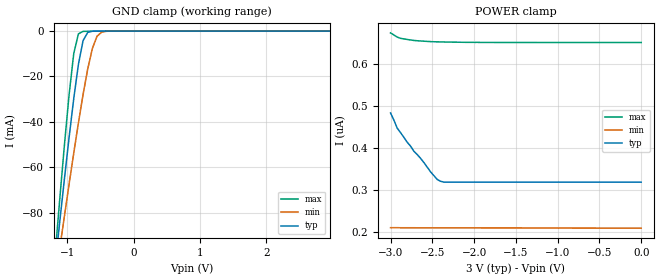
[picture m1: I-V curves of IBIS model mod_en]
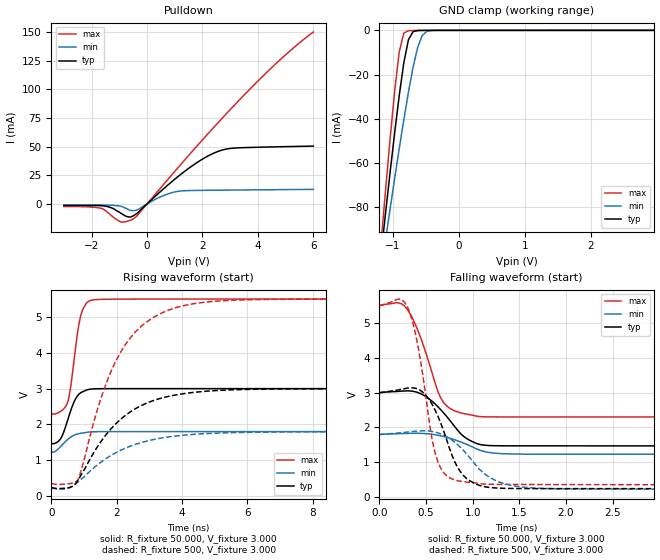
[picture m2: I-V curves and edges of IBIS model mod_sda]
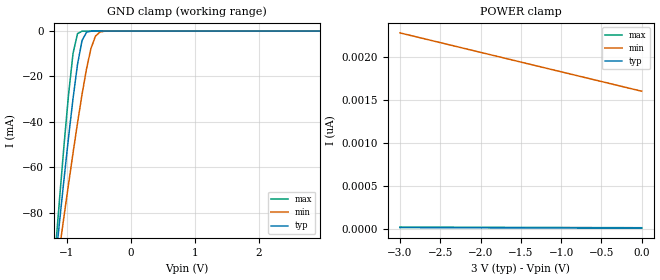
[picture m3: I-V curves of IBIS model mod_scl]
| IBIS (I/O, Buffer, Information, Specification) Model, officially
| electronic behavioral standard for Buffer structures of digital pins.
[IBIS ver]  4.0
[File name] m24c32_tssop8.ibs
[File Rev]  1.0
[Date]   5 April 2013
[Source]   CAD & Design Services (Catania) - STMicroelectronics
[Notes]
   (Note1)  This IBIS model includes the TSSOP8 package data
   (Note2)  This IBIS model has some Notes about the non-monotonicity
   of the I-V curves, but they are not indicative of problems
   inside the model;
[Copyright] (c) 2013 STMicroelectronics
|   Component M24C32
[Component] M24C32
[Manufacturer] STMicroelectronics
[Package]
| variable   typ   min   max
R_pkg   0.0   0.0   0.0
L_pkg   0.0H   0.0H   0.0H
C_pkg   0.0F   0.0F   0.0F
[Pin]  signal_name   model_name   R_pin   L_pin   C_pin
1   E0   mod_en   NA   NA   NA
2   E1   mod_en   NA   NA   NA
3   E2   mod_en   NA   NA   NA
4   VSS   GND   NA   NA   NA
5   SDA   mod_sda   NA   NA   NA
6   SCL   mod_scl   NA   NA   NA
7   WCN   mod_wcn   NA   NA   NA
8   VCC   POWER   NA   NA   NA
[Package Model]  182696_TSSOP8
[Define Package Model]  182696_TSSOP8
[Manufacturer]  STMicroelectronics
[OEM]  STMicroelectronics
[Description]  8 pin TSSOP package
[Number Of Pins]  8
[Pin Numbers]
|Pin Num   Terminal Name
1   | net1
2   | net2
3   | net3
4   | net4_GND
5   | net5
6   | net6
7   | net7
8   | net8_VDD
[Model Data]
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[End Model Data]
[End Package Model]
| Models and submodels in the file (4): mod_en (Input), mod_sda (I/O_open_drain), mod_scl (Input), mod_wcn (Input)
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|   Model mod_en
[Model]   mod_en
Model_type Input
Vinl   =   0.900V
Vinh   =   2.100V
C_comp   2.219pF   2.024pF   2.433pF
[Temperature Range]   25.0000   0.1250k   -40.0000
[Voltage Range]   3.0000V   1.8000V   5.5000V
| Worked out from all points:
|   GND clamp passes 1 mA (typ) near -0.70 V on its own axis
[GND_clamp]
|Voltage   I(typ)   I(min)   I(max)
-3V       -632.3mA   -502.5mA   -782.2mA
-1.18V    -103mA     -110.1mA   -98.28mA
-1.11V    -83.81mA   -95.65mA   -73.74mA
-1.04V    -65mA      -81.41mA   -50.04mA
-970mV    -46.81mA   -67.4mA    -27.99mA
-900mV    -29.69mA   -53.72mA   -9.875mA
-830mV    -14.68mA   -40.49mA   -1.207mA
-760mV    -4.236mA   -27.99mA   -124.1uA
-620mV    -70.96uA   -7.667mA   -43.96uA
-550mV    -18.49uA   -2.282mA   -30.81uA
-480mV    -9.663uA   -457.1uA   -18.98uA
2.95V     1.011uA    747.3nA    5.256uA
[POWER_clamp]
|Voltage   I(typ)   I(min)   I(max)
-3V       483.2nA    210.9nA    673.2nA
-2.92V    447.1nA    210.9nA    663.2nA
-2.8V     413.6nA    210.8nA    657.6nA
-2.76V    404.4nA    210.8nA    656.4nA
-2.72V    392.2nA    210.8nA    655.3nA
-2.68V    384.4nA    210.7nA    654.5nA
-2.6V     365.3nA    210.7nA    653.5nA
-2.52V    343.2nA    210.7nA    652.5nA
-2.44V    325.1nA    210.6nA    652nA
-2.4V     321nA      210.6nA    651.8nA
-2.36V    319nA      210.6nA    651.6nA
0V        319nA      209.8nA    650.4nA
|   Model mod_sda
[Model]   mod_sda
Model_type I/O_open_drain
Polarity   Non-Inverting
Enable   Active-High
Vinl   =   0.900V
Vinh   =   2.100V
Vmeas  =   1.500V
Cref   =   10pF
Rref   =   1k
Vref   =   3.000V
C_comp   2.925pF   2.793pF   3.207pF
[Temperature Range]   25.0000   0.1250k   -40.0000
[Voltage Range]   3.0000V   1.8000V   5.5000V
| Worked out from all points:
|   slope of the pulldown table from 0 to 0.45 V, typ, clamps not added: 44.7 ohm
|   GND clamp passes 1 mA (typ) near -0.70 V on its own axis
|   rising waveform, R_fixture 50.000, V_fixture 3.000: 20-80 % time 357ps typ, 419ps min, 284ps max; typ from 1.47 V to 3 V
|   rising waveform, R_fixture 500, V_fixture 3.000: 20-80 % time 1.55ns typ, 1.71ns min, 1.36ns max; typ from 0.243 V to 3 V
|   falling waveform, R_fixture 50.000, V_fixture 3.000: 20-80 % time 301ps typ, 316ps min, 241ps max; typ from 3 V to 1.47 V
|   falling waveform, R_fixture 500, V_fixture 3.000: 20-80 % time 247ps typ, 351ps min, 184ps max; typ from 3 V to 0.243 V
[Pulldown]
|Voltage   I(typ)   I(min)   I(max)
-3V       -1.423mA   -700uA     -2.3mA
-1.9V     -1.423mA   -747uA     -2.942mA
-1.5V     -1.922mA   -945.3uA   -5.832mA
-900mV    -8.724mA   -2.34mA    -15.92mA
-700mV    -11.22mA   -4.514mA   -15.11mA
-500mV    -10.4mA    -5.884mA   -13.16mA
900mV     19.57mA    9.89mA     25.58mA
1.8V      36.08mA    11.8mA     50.48mA
2.5V      45.28mA    12mA       69.26mA
3.1V      48.68mA    12.14mA    84.88mA
4.3V      49.66mA    12.4mA     114.4mA
6V        50.5mA     12.74mA    150mA
[GND_clamp]
|Voltage   I(typ)   I(min)   I(max)
-3V       -632.3mA   -502.5mA   -782.2mA
-1.18V    -103mA     -110.1mA   -98.29mA
-1.11V    -83.81mA   -95.65mA   -73.75mA
-1.04V    -65mA      -81.41mA   -50.05mA
-970mV    -46.82mA   -67.4mA    -28mA
-900mV    -29.7mA    -53.72mA   -9.899mA
-830mV    -14.69mA   -40.49mA   -1.245mA
-760mV    -4.25mA    -28mA      -159.3uA
-620mV    -83.69uA   -7.672mA   -65.52uA
-550mV    -26.12uA   -2.289mA   -45.81uA
-480mV    -12.79uA   -464.3uA   -27.85uA
2.95V     1.011uA    747.3nA    5.256uA
[Ramp]
| variable   typ   min   max
dV/dt_r  0.9163/0.4218n   0.3404/0.5426n   1.9194/0.3308n
dV/dt_f  0.9163/0.3279n   0.3404/0.3803n   1.9194/0.2635n
R_load = 50.0000
[Rising Waveform]
R_fixture= 50.000
V_fixture= 3.000
V_fixture_min= 1.800
V_fixture_max= 5.500
|time   V(typ)   V(min)   V(max)
0s        1.473V     1.233V     2.301V
270ps     1.586V     1.37V      2.358V
510ps     2.157V     1.589V     2.656V
600ps     2.408V     1.652V     3.115V
720ps     2.679V     1.71V      3.997V
810ps     2.81V      1.737V     4.616V
900ps     2.887V     1.755V     5.043V
1.05ns    2.951V     1.775V     5.357V
1.23ns    2.989V     1.794V     5.469V
15ns      3V         1.8V       5.5V
[Rising Waveform]
R_fixture= 500
V_fixture= 3.000
V_fixture_min= 1.800
V_fixture_max= 5.500
|time   V(typ)   V(min)   V(max)
0s        243.2mV    229.7mV    359.2mV
570ps     245.7mV    236.2mV    349.6mV
795ps     418.2mV    382.8mV    432.2mV
915ps     598mV      474.2mV    728.5mV
1.515ns   1.52V      946.6mV    2.725V
2.055ns   2.091V     1.25V      3.911V
2.685ns   2.496V     1.477V     4.686V
3.6ns     2.787V     1.653V     5.196V
5.805ns   2.974V     1.776V     5.475V
15ns      3V         1.8V       5.5V
[Falling Waveform]
R_fixture= 50.000
V_fixture= 3.000
V_fixture_min= 1.800
V_fixture_max= 5.500
|time   V(typ)   V(min)   V(max)
0s        3V         1.8V       5.5V
195ps     3.036V     1.821V     5.583V
270ps     3.049V     1.827V     5.486V
420ps     2.996V     1.833V     4.737V
630ps     2.588V     1.777V     3.015V
690ps     2.415V     1.741V     2.713V
900ps     1.753V     1.555V     2.403V
1.08ns    1.511V     1.344V     2.313V
1.68ns    1.473V     1.234V     2.302V
15ns      1.473V     1.233V     2.301V
[Falling Waveform]
R_fixture= 500
V_fixture= 3.000
V_fixture_min= 1.800
V_fixture_max= 5.500
|time   V(typ)   V(min)   V(max)
0s        3V         1.8V       5.5V
210ps     3.081V     1.844V     5.687V
300ps     3.129V     1.869V     5.465V
405ps     3.111V     1.896V     4.457V
600ps     2.485V     1.866V     1.241V
720ps     1.657V     1.738V     617.8mV
900ps     625.9mV    1.345V     445.3mV
1.23ns    266.7mV    498.4mV    367.5mV
1.8ns     245.2mV    247.4mV    362mV
15ns      243.2mV    229.7mV    359.2mV
|   Model mod_scl
[Model]   mod_scl
Model_type Input
Vinl   =   0.900V
Vinh   =   2.100V
C_comp   2.219pF   2.024pF   2.433pF
[Temperature Range]   25.0000   0.1250k   -40.0000
[Voltage Range]   3.0000V   1.8000V   5.5000V
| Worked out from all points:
|   GND clamp passes 1 mA (typ) near -0.70 V on its own axis
[GND_clamp]
|Voltage   I(typ)   I(min)   I(max)
-3V       -632.3mA   -502.5mA   -782.2mA
-1.18V    -103mA     -110mA     -98.27mA
-1.11V    -83.8mA    -95.64mA   -73.72mA
-1.04V    -64.99mA   -81.4mA    -50.02mA
-970mV    -46.8mA    -67.39mA   -27.96mA
-900mV    -29.68mA   -53.7mA    -9.828mA
-830mV    -14.66mA   -40.48mA   -1.131mA
-760mV    -4.202mA   -27.98mA   -52.91uA
-620mV    -46.95uA   -7.639mA   -90.25nA
-550mV    -3.894uA   -2.251mA   -3.716nA
-480mV    -321.5nA   -432.2uA   -153.9pA
2.95V     6.148pA    1.861nA    6.002pA
[POWER_clamp]
|Voltage   I(typ)   I(min)   I(max)
-3V       13.21pA    2.28nA     18.37pA
-1.68V    10.04pA    1.981nA    15.23pA
-600mV    7.58pA     1.737nA    12.78pA
0V        6.257pA    1.601nA    11.44pA
